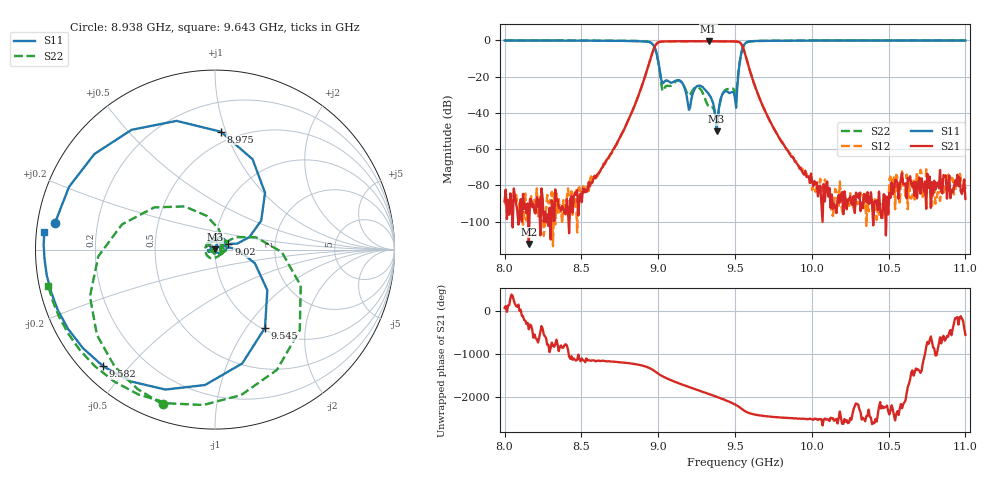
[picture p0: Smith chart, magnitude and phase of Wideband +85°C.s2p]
!Agilent Technologies,N5230C,MY49001174,A.09.42.22
!Agilent N5230C: A.09.42.22
!Date: Friday, February 13, 2026 12:48:19
!Correction: S11(Full 2 Port(1,2))
!S21(Full 2 Port(1,2))
!S12(Full 2 Port(1,2))
!S22(Full 2 Port(1,2))
!S2P File: Measurements: S11, S21, S12, S22:
# Hz S  dB  R 50
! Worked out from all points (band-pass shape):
!   401 points, 8 GHz to 11 GHz, reference 50 ohm
!   highest |S21| = -0.51 dB at 9.328 GHz (marker M1); lowest = -112.3 dB at 8.158 GHz (marker M2)
!   |S21| within 3 dB of the highest: 8.978 GHz to 9.549 GHz (571 MHz wide, 6.16 % of centre)
!   lowest |S11| = -50.2 dB at 9.38 GHz (marker M3), VSWR 1.01, Z = 49.8 + j0.264 ohm
!   |S11| at or under -10 dB: 8.997 GHz to 9.535 GHz (538.3 MHz wide, 5.81 % of centre)
!   |S22| runs from -46.5 to -0.1 dB; largest |S21 - S12| = 0.0016
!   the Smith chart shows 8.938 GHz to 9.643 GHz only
!   S11 on the Smith chart (normalised r, x): 8.938 GHz: 0.05, +0.08; 8.975 GHz: 0.41, +0.96; 9.02 GHz: 1.16, +0.07; 9.545 GHz: 1.03, -1.23; 9.582 GHz: 0.06, -0.43; 9.643 GHz: 0.02, +0.05
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8e9  -0.14 73.0  -88.79 66.8  -88.57 -133.8  -0.16 86.5
8.1575e9  -0.14 59.6  -112.32 -67.8  -97.25 -16.2  -0.15 73.7
8.5025e9  -0.17 19.3  -89.28 -29.2  -84.02 -34.3  -0.18 37.6
8.7125e9  -0.27 -26.3  -59.87 -104.6  -59.40 -104.5  -0.23 1.7
8.84e9  -0.43 -84.4  -37.38 -154.2  -37.37 -154.0  -0.34 -38.3
8.9375e9  -0.88 170.5  -13.66 117.6  -13.65 117.6  -0.82 -108.8
8.975e9  -3.64 87.2  -4.06 41.3  -4.05 41.2  -3.72 -176.7
9.005e9  -13.83 19.9  -1.00 -35.1  -1.00 -35.1  -14.23 104.0
9.02e9  -21.80 22.7  -0.74 -67.5  -0.74 -67.5  -23.82 45.8
9.08e9  -23.29 49.2  -0.60 -169.7  -0.60 -169.7  -25.18 146.0
9.1475e9  -22.55 15.8  -0.55 95.2  -0.55 95.2  -22.84 8.5
9.23e9  -28.21 135.3  -0.51 -10.7  -0.52 -10.7  -26.95 15.5
9.3275e9  -29.37 72.5  -0.51 -132.2  -0.51 -132.1  -36.19 -177.6
9.38e9  -50.18 121.3  -0.53 160.3  -0.52 160.4  -46.50 -8.5
9.44e9  -28.07 -176.2  -0.58 77.5  -0.57 77.5  -27.22 129.4
9.5e9  -32.07 176.5  -0.69 -19.9  -0.67 -19.9  -29.02 -23.6
9.545e9  -5.73 -57.4  -2.68 -125.4  -2.67 -125.3  -5.71 -22.8
9.5825e9  -0.91 -133.8  -12.57 153.3  -12.56 153.3  -0.96 -107.0
9.6425e9  -0.39 174.0  -28.26 96.3  -28.25 96.3  -0.44 -167.6
1.00025e10  -0.16 86.1  -78.20 -8.3  -82.64 30.6  -0.18 90.9
1.0505e10  -0.11 40.2  -84.32 108.0  -76.70 96.2  -0.14 41.1
1.1e10  -0.12 8.8  -87.54 159.4  -81.96 152.5  -0.16 8.3
